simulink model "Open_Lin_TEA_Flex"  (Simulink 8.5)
settings: Solver=ode113  StartTime=0.0  StopTime=100000  RelTol=1e-3
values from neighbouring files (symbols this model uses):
  Kpqr = lqr(sys,Q0,R0)    [des.m]
  wo = 0.0011    [start.m]    (also in start1.m; start2.m; start3.m)
undefined symbols (not defined in the file or in its folder): Af, Bf, Cf, Df

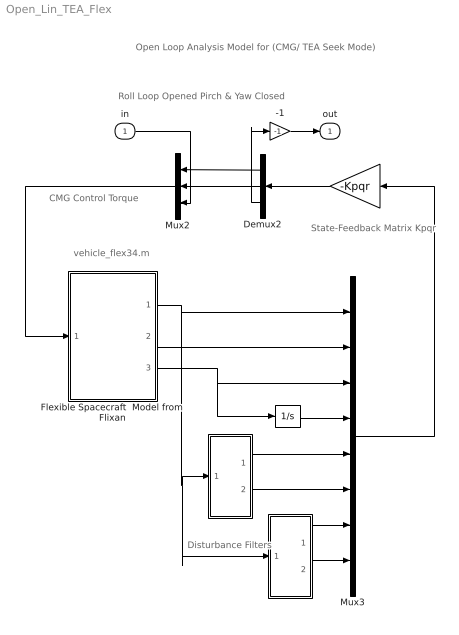
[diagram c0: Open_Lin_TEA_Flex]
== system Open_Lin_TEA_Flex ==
  note: Open Loop Analysis Model for (CMG/ TEA Seek Mode)
  note: CMG Control Torque
  note: State-Feedback Matrix Kpqr
  note: Roll Loop Opened Pirch & Yaw Closed
  note: vehicle_flex34.m
  note: Disturbance Filters
  in : Inport  PortDimensions=1
  " " : Gain  Gain=-Kpqr  Multiplication=Matrix(K*u)
  "  " : Integrator
  "   " : Subsystem
  "    " : Subsystem
  -1 : Gain  Gain=-1
  Demux2 : Demux  Outputs=3
  Flexible Spacecraft  Model from Flixan : Subsystem
  Mux2 : Mux  Inputs=3
  Mux3 : Mux  Inputs=[3, 3, 3, 3, 1, 1, 1, 1]
  out : Outport
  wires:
  Mux2/1 -> Flexible Spacecraft  Model from Flixan/1(Tcmg)
  -1/1 -> out/1
  Flexible Spacecraft  Model from Flixan/3("Hcmg ") -> Mux3/3, "  "/1
  Flexible Spacecraft  Model from Flixan/1(att-lv) -> "    "/1(psi), "   "/1(the), Mux3/1
  Flexible Spacecraft  Model from Flixan/2(w-lv) -> Mux3/2
  "  "/1 -> Mux3/4
  "    "/1(b1) -> Mux3/7
  "    "/2(b2) -> Mux3/8
  "   "/2(a2) -> Mux3/6
  "   "/1(a1) -> Mux3/5
  " "/1 -> Demux2/1
  Mux3/1 -> " "/1
  Demux2/1 -> Mux2/1
  Demux2/2 -> Mux2/2
  in/1 -> Mux2/3
  Demux2/3 -> -1/1

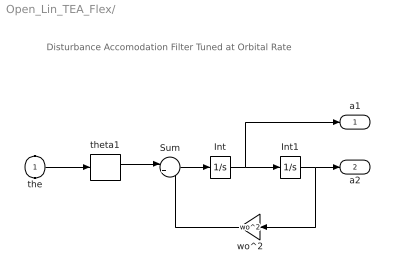
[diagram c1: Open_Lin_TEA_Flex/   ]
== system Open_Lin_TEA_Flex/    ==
  note: Disturbance Accomodation Filter Tuned at Orbital Rate
  the : Inport
  Int : Integrator
  Int1 : Integrator
  Sum : Sum  Inputs=|+-
  theta1 : Selector  InputPortWidth=3  Indices=[2]
  wo^2 : Gain  Gain=wo^2
  a1 : Outport
  a2 : Outport  Port=2
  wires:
  the/1 -> theta1/1
  theta1/1 -> Sum/1
  wo^2/1 -> Sum/2
  Int1/1 -> a2/1, wo^2/1
  Sum/1 -> Int/1
  Int/1 -> a1/1, Int1/1

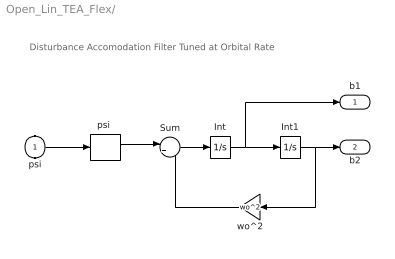
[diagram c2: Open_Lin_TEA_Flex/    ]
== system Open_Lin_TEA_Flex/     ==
  note: Disturbance Accomodation Filter Tuned at Orbital Rate
  psi : Inport
  Int : Integrator
  Int1 : Integrator
  Sum : Sum  Inputs=|+-
  "psi " : Selector  InputPortWidth=3  Indices=[3]
  wo^2 : Gain  Gain=wo^2
  b1 : Outport
  b2 : Outport  Port=2
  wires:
  psi/1 -> "psi "/1
  "psi "/1 -> Sum/1
  wo^2/1 -> Sum/2
  Int1/1 -> b2/1, wo^2/1
  Sum/1 -> Int/1
  Int/1 -> b1/1, Int1/1

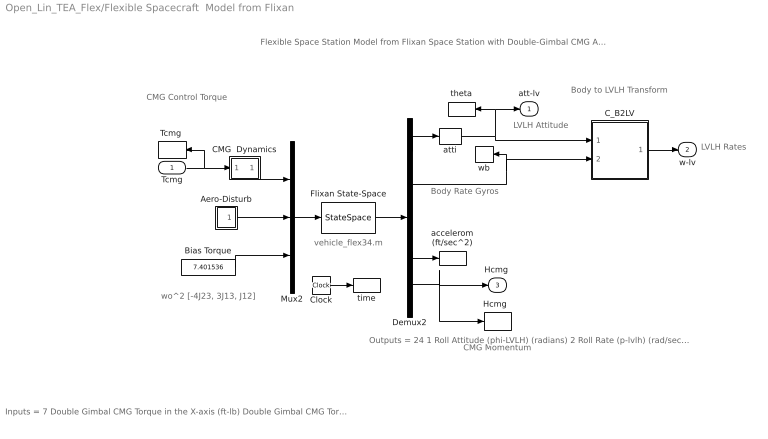
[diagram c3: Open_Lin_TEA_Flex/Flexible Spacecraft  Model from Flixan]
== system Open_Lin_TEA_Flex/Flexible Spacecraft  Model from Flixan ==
  note: wo^2 [-4J23, 3J13, J12]
  note: CMG Momentum
  note: LVLH Rates
  note: CMG Control Torque
  note: Outputs = 24 1 Roll Attitude (phi-LVLH) (radians) 2 Roll Rate (p-lvlh) (rad/sec) 3 Pitch Attitude (thet-LVLH) (radians) 4 Pitch Rate (q-lvlh) (rad/sec) 5 Yaw Attitude (psi-LVLH) (radians) 6 Yaw Rate (r-lvlh) (rad/sec) 7 Angle of attack, alfa, (radians) 8 Angle of sideslip, beta, (radian) 9 Change in Altitude, delta-h, (feet) 10 Forward Acceleration (V-dot) (ft/sec) 11 Cross Range Velocity (Vcr) (ft/sec) 12 Rate-Gyro # 1, Roll Rate (Body) (rad/sec) 13 Rate-Gyro # 2, Pitch Rate (Body) (rad/sec) 14 Rate-Gyro # 3, Yaw Rate (Body) (rad/sec) 15 Gyro # 4, Roll Attitude (Body) (radians) 16 Gyro # 5, Pitch Attitude (Body) (radians) 17 Gyro # 6, Yaw Attitude (Body) (radians) 18 Accelerom # 1, (along X), (ft/sec^2) Translat. Accelerat. 19 Accelerom # 2, (along Z), (ft/sec^2) Translat. Accelerat. 20 Accelerom # 3, (along X), (ft/sec^2) Translat. Accelerat. 21 Accelerom # 4, (along Z), (ft/sec^2) Translat. Accelerat. 22 Double Gimbal CMG Momentum Change in X-axis (ft-lb-sec) 23 Double Gimbal CMG Momentum Change in Y-axis (ft-lb-sec) 24 Double Gimbal CMG Momentum Change in Z-axis (ft-lb-sec)
  note: Inputs = 7 Double Gimbal CMG Torque in the X-axis (ft-lb) Double Gimbal CMG Torque in the Y-axis (ft-lb) Double Gimbal CMG Torque in the Z-axis (ft-lb) External Torque Input 1 (ft-lb), direct: External Torque Input 2 (ft-lb), direct: External Torque Input 3 (ft-lb), direct: Ext Torque Direct.=(0.197, -0.5964, -0.7782)
  note: Flexible Space Station Model from Flixan Space Station with Double-Gimbal CMG Array (Flex)
  note: Body Rate Gyros
  note: LVLH Attitude
  note: Body to LVLH Transform
  note: vehicle_flex34.m
  Tcmg : Inport  PortDimensions=3
  Aero-Disturb : Subsystem
  Bias Torque : Constant  Value=7.401536
  CMG  Dynamics : Subsystem
  C_B2LV : Subsystem
  Clock : Clock
  Demux2 : Demux  Outputs=[11, 3, 3, 4, 3]
  Flixan State-Space : StateSpace  A=Af  B=Bf  C=Cf  D=Df  X0=0
  "Hcmg  " : ToWorkspace  VariableName=Hcmg  SampleTime=-1
  Mux2 : Mux  Inputs=[3, 3, 1]
  "Tcmg " : ToWorkspace  VariableName=Tcmg  SampleTime=-1
  accelerom (ft/sec^2) : ToWorkspace  VariableName=accel  SampleTime=-1
  atti : Selector  InputPortWidth=11  Indices=[1 3 5]
  theta : ToWorkspace  VariableName=theta  SampleTime=-1
  time : ToWorkspace  VariableName=time  SampleTime=-1
  wb : ToWorkspace  VariableName=wb  SampleTime=-1
  att-lv : Outport
  w-lv : Outport  Port=2
  "Hcmg " : Outport  Port=3
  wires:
  Mux2/1 -> Flixan State-Space/1
  Flixan State-Space/1 -> Demux2/1
  Bias Torque/1 -> Mux2/3
  Clock/1 -> time/1
  Demux2/5 -> "Hcmg  "/1, "Hcmg "/1
  Demux2/1 -> atti/1
  Demux2/4 -> accelerom (ft/sec^2)/1
  Tcmg/1 -> CMG  Dynamics/1(I), "Tcmg "/1
  Aero-Disturb/1(Td) -> Mux2/2
  CMG  Dynamics/1(O) -> Mux2/1
  atti/1 -> theta/1, att-lv/1, C_B2LV/1(atti)
  C_B2LV/1(wlv) -> w-lv/1
  Demux2/2 -> wb/1, C_B2LV/2(wb)

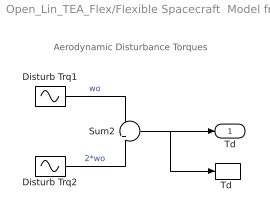
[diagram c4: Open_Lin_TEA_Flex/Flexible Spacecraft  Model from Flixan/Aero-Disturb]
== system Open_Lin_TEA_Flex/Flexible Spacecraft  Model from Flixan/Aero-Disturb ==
  note: Aerodynamic Disturbance Torques
  Disturb Trq1 : Sin  Amplitude=[1, 3, 1]  Bias="[1  8  1]"  Frequency=[wo, wo, wo]  SampleTime=0
  Disturb Trq2 : Sin  Amplitude=[1, 1, 1]*0.5  Frequency=[wo, wo, wo]*2  SampleTime=0
  Sum2 : Sum  Inputs=+|+
  "Td " : ToWorkspace  VariableName=Td  SampleTime=-1
  Td : Outport
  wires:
  Disturb Trq1/1 -> Sum2/1  "wo"
  Sum2/1 -> Td/1, "Td "/1
  Disturb Trq2/1 -> Sum2/2  "2*wo"

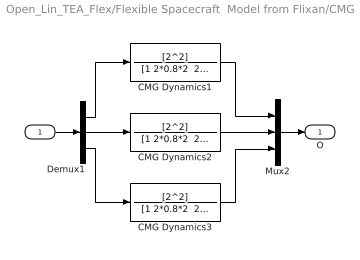
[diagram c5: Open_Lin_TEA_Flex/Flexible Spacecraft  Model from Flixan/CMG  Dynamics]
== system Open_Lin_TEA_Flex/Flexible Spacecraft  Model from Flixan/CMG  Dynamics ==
  I : Inport
  CMG Dynamics1 : TransferFcn  Numerator=[2^2]  Denominator="[1 2*0.8*2  2^2]"
  CMG Dynamics2 : TransferFcn  Numerator=[2^2]  Denominator="[1 2*0.8*2  2^2]"
  CMG Dynamics3 : TransferFcn  Numerator=[2^2]  Denominator="[1 2*0.8*2  2^2]"
  Demux1 : Demux  Outputs=3
  Mux2 : Mux  Inputs=3
  O : Outport
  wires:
  Mux2/1 -> O/1
  I/1 -> Demux1/1
  Demux1/3 -> CMG Dynamics3/1
  Demux1/1 -> CMG Dynamics1/1
  Demux1/2 -> CMG Dynamics2/1
  CMG Dynamics1/1 -> Mux2/1
  CMG Dynamics3/1 -> Mux2/3
  CMG Dynamics2/1 -> Mux2/2

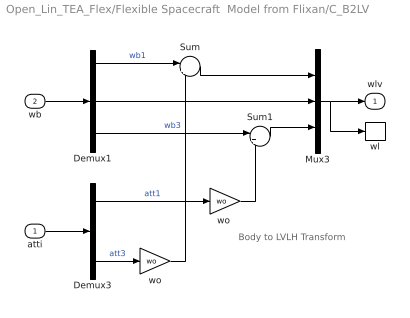
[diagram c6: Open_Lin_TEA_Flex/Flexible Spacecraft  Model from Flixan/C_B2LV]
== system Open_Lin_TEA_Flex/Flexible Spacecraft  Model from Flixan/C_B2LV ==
  note: Body to LVLH Transform
  atti : Inport  PortDimensions=3
  wb : Inport  Port=2  PortDimensions=3
  Demux1 : Demux  Outputs=3
  Demux3 : Demux  Outputs=3
  Mux3 : Mux  Inputs=3
  Sum : Sum  Inputs=|++
  Sum1 : Sum  Inputs=|+-
  wl : ToWorkspace  VariableName=wl  SampleTime=-1
  wo : Gain  Gain=wo
  "wo " : Gain  Gain=wo
  wlv : Outport
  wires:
  "wo "/1 -> Sum1/2
  Demux1/3 -> Sum1/1  "wb3"
  wo/1 -> Sum/2
  Demux1/2 -> Mux3/2
  Demux3/1 -> "wo "/1  "att1"
  Mux3/1 -> wl/1, wlv/1
  wb/1 -> Demux1/1
  atti/1 -> Demux3/1
  Sum1/1 -> Mux3/3
  Demux3/3 -> wo/1  "att3"
  Sum/1 -> Mux3/1
  Demux1/1 -> Sum/1  "wb1"
